FUNCTION_BLOCK FB_Command
VAR_INPUT
	bEnable				:	BOOL;
	bEnPos				:	BOOL;
	bEnNeg				:	BOOL;
	fOverride			:	LREAL;
	bGearIn				:	BOOL;
	bCamIn				:	BOOL;
	nMasterAxisId		:	UINT;
	bGearOut			:	BOOL;
	bCamOut				:	BOOL;
	bJogFwd				:	BOOL;
	bJogBwd				:	BOOL;
	bReset				:	BOOL;
	bStop				:	BOOL;
	bRun				:	BOOL;
	fPosition			:	LREAL;
	fVelocity			:	LREAL;
	fRatio				:	LREAL := 1.0;
	nCamTableID			:	UDINT := 1;
	nPtpMode			:	USINT;
	
	
	
	
	
END_VAR
VAR_OUTPUT
END_VAR
VAR
END_VAR

END_FUNCTION_BLOCK
